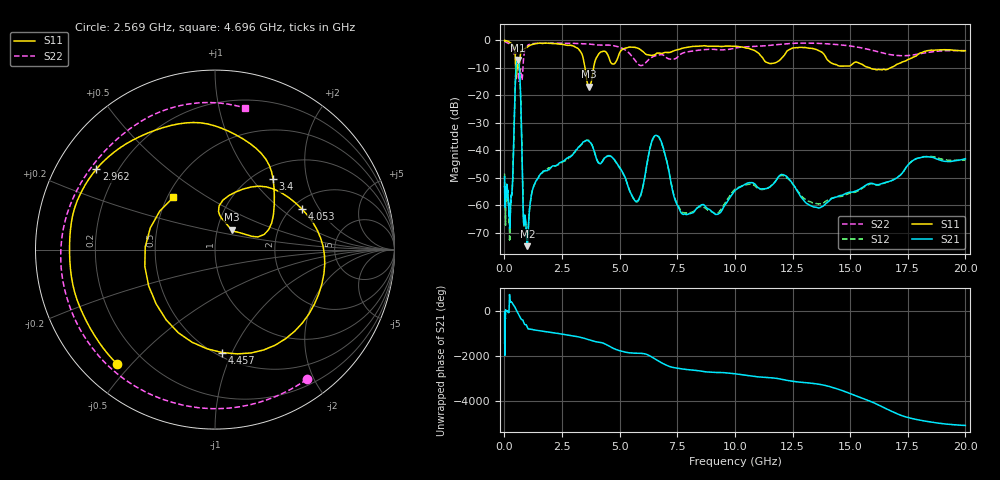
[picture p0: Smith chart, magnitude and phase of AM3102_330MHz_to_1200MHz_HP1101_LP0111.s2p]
! Date/Time: Tue, Sep 11, 2018 5:22 PM
! Network Analyzer: Agilent Technologies E8362B Rev: A.07.50.63
! Sweep from 0.010 to 20.000 GHz, 1601 Points, Sweep Type: LOG
! Power Supply: 4.949 V, 0.001 A
# Hz S DB R 50
!freq MagS11 AngS11 MagS21 AngS21 MagS12 AngS12 MagS22 AngS22
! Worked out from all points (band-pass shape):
!   1601 points, 10 MHz to 20 GHz, reference 50 ohm
!   highest |S21| = -7.16 dB at 594.7 MHz (marker M1); lowest = -74.8 dB at 998.1 MHz (marker M2)
!   |S21| within 3 dB of the highest: 503.7 MHz to 653.5 MHz (149.8 MHz wide, 25.9 % of centre)
!   lowest |S11| = -16.9 dB at 3.668 GHz (marker M3), VSWR 1.34, Z = 58.6 + j13.2 ohm
!   |S11| at or under -10 dB: 487.1 MHz to 546.2 MHz (59.15 MHz wide, 11.4 % of centre); 3.5 GHz to 3.869 GHz (369.1 MHz wide, 10 % of centre); 15.86 GHz to 16.75 GHz (887.8 MHz wide, 5.45 % of centre)
!   |S22| runs from -14.9 to -0.2 dB; largest |S21 - S12| = 0.0063
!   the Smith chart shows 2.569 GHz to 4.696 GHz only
!   S11 on the Smith chart (normalised r, x): 2.569 GHz: 0.11, -0.45; 2.962 GHz: 0.12, +0.30; 3.4 GHz: 1.21, +1.29; 4.053 GHz: 2.25, +1.43; 4.457 GHz: 0.54, -0.92; 4.696 GHz: 0.54, +0.36
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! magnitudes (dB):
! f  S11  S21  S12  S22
! 10 MHz  0.0  -49.6  -48.4  -0.2
! 35.55 MHz  -0.1  -58.7  -59.7  -0.4
! 126.4 MHz  -0.2  -53.6  -55.3  -0.9
! 230 MHz  -0.7  -68.1  -72.2  -1.3
! 354.3 MHz  -1.7  -51.9  -52.6  -3.5
! 447.2 MHz  -3.6  -22.8  -22.8  -4.3
! 594.7 MHz  -9.0  -7.2  -7.3  -10.5
! 695.6 MHz  -4.9  -17.9  -17.9  -10.4
! 833.3 MHz  -3.2  -65.9  -66.1  -6.6
! 998.1 MHz  -2.4  -74.8  -71.9  -1.9
! 1.59 GHz  -1.1  -48.4  -48.4  -1.0
! 2.569 GHz  -1.5  -44.0  -44.0  -1.1
! 2.962 GHz  -2.0  -41.6  -41.4  -1.1
! 3.4 GHz  -5.9  -37.1  -37.3  -1.2
! 3.668 GHz  -16.9  -36.7  -36.4  -1.3
! 4.053 GHz  -5.4  -44.3  -44.0  -1.7
! 4.457 GHz  -4.8  -42.2  -42.0  -1.7
! 4.696 GHz  -8.6  -42.7  -42.8  -1.9
! 5.652 GHz  -2.5  -58.2  -58.2  -7.1
! 6.58 GHz  -4.8  -34.5  -34.7  -5.5
! 7.92 GHz  -2.5  -63.3  -62.8  -4.2
! 20 GHz  -3.8  -43.0  -43.5  -3.7
